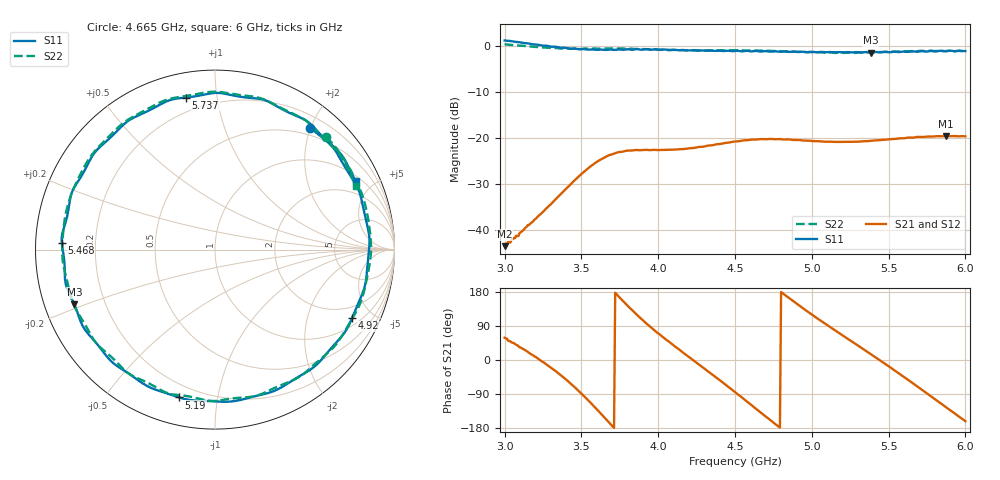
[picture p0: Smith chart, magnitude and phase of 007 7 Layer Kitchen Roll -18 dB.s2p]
!  04/11/2025  14:50:58
! Ref Plane: 0.000 mm
# MHZ S MA R  50
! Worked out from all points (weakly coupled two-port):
!   401 points, 3 GHz to 6 GHz, reference 50 ohm
!   highest |S21| = -19.62 dB at 5.872 GHz (marker M1); lowest = -43.5 dB at 3 GHz (marker M2)
!   lowest |S11| = -1.5 dB at 5.385 GHz (marker M3), VSWR 11.56, Z = 4.48 - j9.3 ohm
!   |S11| at or under -10 dB: nowhere
!   |S22| runs from -1.6 to 0.3 dB; largest |S21 - S12| = 0.0023
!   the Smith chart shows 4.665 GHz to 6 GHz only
!   S11 on the Smith chart (normalised r, x): 4.665 GHz: 0.38, +2.00; 4.92 GHz: 1.34, -3.78; 5.19 GHz: 0.13, -0.78; 5.468 GHz: 0.08, +0.02; 5.737 GHz: 0.12, +0.82; 6 GHz: 1.26, +3.98
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3000  1.136 -112.8  0.006697 58.7  0.006767 60.2  1.034 -116.9
3270  0.9977 179.3  0.01715 -11.0  0.01699 -9.1  0.9511 175.6
3390  0.9491 141.6  0.02701 -48.0  0.0271 -47.5  0.9315 137.4
3502.5  0.9147 99.2  0.04089 -89.6  0.04086 -89.0  0.9211 94.9
3607.5  0.8985 54.6  0.05592 -133.0  0.05608 -132.7  0.9228 50.9
3735  0.9056 -2.1  0.06952 170.9  0.06983 172.1  0.9285 -4.9
3870  0.9124 -56.7  0.0736 115.9  0.07427 117.2  0.9197 -59.3
4005  0.8998 -104.0  0.0738 68.9  0.07366 69.7  0.9011 -105.9
4245  0.8836 -178.8  0.07838 -5.8  0.0787 -4.6  0.8855 179.7
4357.5  0.8768 147.4  0.08341 -40.0  0.08383 -38.8  0.8896 145.0
4500  0.8745 102.9  0.09124 -84.9  0.09202 -84.1  0.8862 99.1
4665  0.8608 51.9  0.09679 -137.6  0.09712 -137.0  0.8819 45.3
4792.5  0.857 12.1  0.09696 -178.3  0.09708 -177.3  0.8694 4.0
4920  0.8538 -26.6  0.09468 143.2  0.09475 144.1  0.8558 -35.0
5002.5  0.8552 -50.3  0.09233 119.3  0.09241 120.1  0.8489 -58.5
5190  0.8476 -103.6  0.09033 67.9  0.09034 68.6  0.8414 -109.6
5385  0.8408 -158.8  0.09284 15.3  0.09333 16.2  0.8444 -161.6
5467.5  0.8547 177.5  0.09533 -7.6  0.09576 -7.0  0.8511 175.7
5505  0.8443 167.4  0.09639 -17.6  0.09704 -16.7  0.8559 165.6
5737.5  0.8626 100.8  0.1027 -84.6  0.1037 -83.5  0.8708 100.3
5872.5  0.867 61.8  0.1045 -124.3  0.1053 -123.3  0.8719 61.1
6000  0.8714 25.9  0.1038 -161.5  0.1043 -160.8  0.8617 24.2
